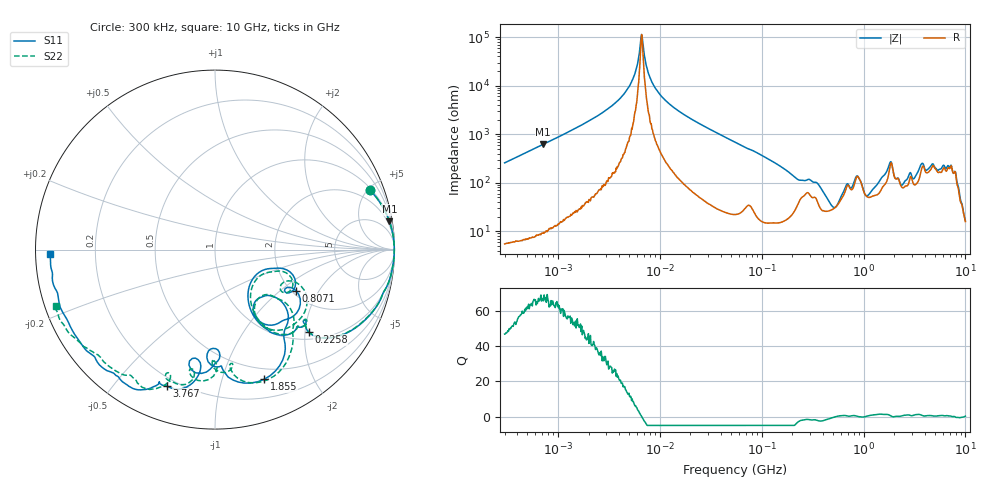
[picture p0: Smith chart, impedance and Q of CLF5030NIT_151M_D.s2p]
! S-Parameter Data Generated by TDK Corporation
! Copyright(C) 2019 TDK Corporation.
! All Rights Reserved.
! TDK P/N: CLF5030NIT-151M-D (Inductor)
! Property: L=150uH at 100kHz
! Size(LxWxT): 5.3x5x2.7mm
! Model Type: s2p (Touchstone File Format Version 1.0)
! Frequency: DC=Yes Start=0.3MHz Stop=10000MHz 802points Log-sweep
! Model Generated on May 10, 2019
! Port Assignments:
!  1 ---@@@--- 2
! Applicable Conditions:
!  Temperature = 25 degC
!  DC Bias Current = 0 A
!  Small Signal Operation
! Terms and conditions regarding TDK Simulation Models
! (1)This simulation model is being provided solely for informational purposes. Please refer to the specifications of the products in terms of detailed characteristics of such products.
! (2)In no event shall TDK Corporation of any of its subsidiaries be liable for any loss or damage arising, directly or indirectly,
!  From any information contained in this simulation model, including, but not limited to loss or damages arising from any inaccuracies, omissions or errors in connection with such information.
! (3)Any and all copyrights on this simulation model are owned by TDK Corporation.
!  Duplication or redistribution of this simulation model without prior written permission from TDK Corporation is prohibited.
! (4)This simulation model is subject to any modification or change without any prior notice.
! (5)Neither TDK Corporation nor any of its subsidiaries shall make any warranty, express or implied,
!  Including but not limited to the correctness, implied warranties of merchantability and fitness for a particular purpose with respect to this simulation models.
! (6)The use of this simulation model shall be deemed to have consented to the terms and conditions hereof.
# Hz S MA R 50
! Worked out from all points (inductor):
!   801 points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, 300 kHz to 10 GHz, reference 50 ohm
!   read as one part in series: L = 136 uH near 318.3 kHz
!   highest Q = 67.1 at 715.8 kHz (marker M1), where L = 137 uH
!   self-resonance near 6.642 MHz
!   S11 on the Smith chart (normalised r, x): 300 kHz: 1.12, +5.14; 225.8 MHz: 1.18, -2.09; 807.1 MHz: 2.11, -1.30; 1.855 GHz: 0.38, -1.38; 3.767 GHz: 0.16, -0.70; 10 GHz: 0.04, -0.01
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300000  0.9248 21.1  0.3602 -67.7  0.3601 -67.7  0.9246 21.1
715804  0.9843 9.2  0.1599 -80.0  0.1599 -79.9  0.9844 9.2
1713600  0.9964 3.6  0.06422 -85.3  0.06419 -85.2  0.9965 3.6
4611084  0.999 0.6  0.01339 -85.6  0.01338 -85.7  0.9991 0.6
5698586  0.9991 0.1  0.005677 -80.7  0.005659 -81.5  0.9991 0.1
6642044  0.9992 -0.3  0.0008794 -4.8  0.0008195 -6.4  0.9992 -0.3
7771787  0.999 -0.6  0.005715 80.5  0.005683 80.4  0.9992 -0.6
9671944  0.9989 -1.2  0.01373 84.6  0.01373 84.6  0.9989 -1.2
5.477226e7  0.9849 -10.5  0.1436 77.6  0.1436 77.6  0.9849 -10.5
2.257919e8  0.695 -41.4  0.5516 32.4  0.5516 32.4  0.6919 -41.2
3.126428e8  0.6404 -42.5  0.5422 22.6  0.5421 22.6  0.6415 -42.0
5.414944e8  0.2698 -41.9  0.7388 -14.9  0.7387 -14.9  0.2863 -41.1
8.070667e8  0.5066 -26.9  0.502 -41.0  0.502 -41.0  0.4906 -22.1
1.085776e9  0.3853 -56.4  0.616 -35.8  0.6159 -35.8  0.3859 -55.1
1.371335e9  0.4485 -37.9  0.5563 -68.1  0.5561 -68.1  0.4768 -37.1
1.767019e9  0.7219 -58.5  0.2698 -94.7  0.2696 -94.7  0.759 -60.2
1.854885e9  0.7726 -69.2  0.1973 -79.8  0.1972 -79.8  0.7812 -70.5
2.477118e9  0.5592 -88.4  0.3661 -92.4  0.3656 -92.4  0.615 -90.3
3.766866e9  0.8056 -109.4  0.1117 -123.7  0.1119 -123.4  0.7765 -108.5
5.526371e9  0.8925 -128.2  0.09595 -140.9  0.09581 -140.2  0.8619 -125.8
7.652089e9  0.9121 -154.9  0.03515 -137.6  0.03593 -137.5  0.9331 -149.3
1e10  0.9178 -178.6  0.04453 -96.6  0.04455 -97.0  0.9392 -160.5
